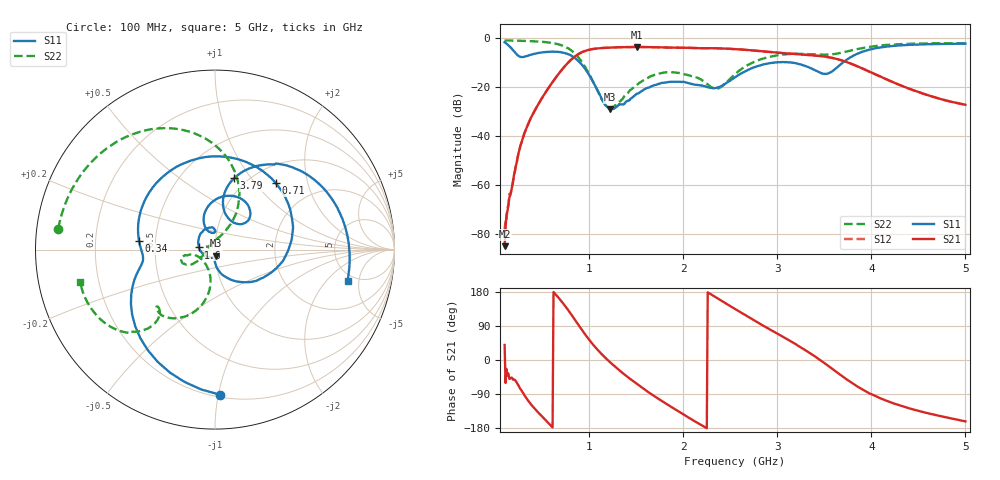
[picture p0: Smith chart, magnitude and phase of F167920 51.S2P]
!  2-Port S-parameters saved by WinCal
! VAR MeasName=S-Parameters (CALIBRATED_DATA) read from VNA (N5242A)
! VAR MeasDate=2016-11-22 9:58:02
! VAR NAME=F167920 51
! VAR FILENAME=F167920 51.S2P
! VAR DATE=2016-11-22 9:58:02
! VAR PHYS_PORTS=1,2
# Hz S DB R 50
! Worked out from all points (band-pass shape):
!   491 points, 100 MHz to 5 GHz, reference 50 ohm
!   highest |S21| = -3.75 dB at 1.51 GHz (marker M1); lowest = -85.1 dB at 100 MHz (marker M2)
!   |S21| within 3 dB of the highest: 881.8 MHz to 3.222 GHz (2.34 GHz wide, 114 % of centre)
!   lowest |S11| = -29.2 dB at 1.22 GHz (marker M3), VSWR 1.07, Z = 50.4 - j3.47 ohm
!   |S11| at or under -10 dB: 897.7 MHz to 3.007 GHz (2.109 GHz wide, 108 % of centre); 3.116 GHz to 3.702 GHz (586 MHz wide, 17.2 % of centre)
!   |S22| runs from -28.7 to -1.1 dB; largest |S21 - S12| = 0.0015
!   S11 on the Smith chart (normalised r, x): 100 MHz: 0.22, -1.01; 340 MHz: 0.40, +0.05; 710 MHz: 1.30, +1.29; 1.6 GHz: 0.83, +0.02; 3.79 GHz: 0.87, +0.83; 5 GHz: 4.33, -3.53
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1e8  -1.84 -88.0  -85.14 39.8  -78.36 -52.7  -1.10 172.4
1.8e8  -4.62 -141.7  -60.63 -47.2  -60.76 -55.6  -1.15 166.3
2.6e8  -7.68 -169.4  -45.45 -73.6  -45.32 -72.4  -1.22 159.9
3.4e8  -7.40 173.5  -36.17 -103.6  -36.14 -103.3  -1.32 153.1
5.5e8  -5.79 104.9  -21.47 -162.2  -21.46 -162.2  -1.84 131.0
7.1e8  -5.99 47.7  -13.00 153.2  -13.00 153.2  -3.13 106.2
8.1e8  -7.32 7.4  -8.85 119.7  -8.86 119.8  -5.21 86.2
9.2e8  -10.83 -37.4  -5.91 80.3  -5.91 80.3  -9.84 65.1
1.07e9  -20.15 -84.8  -4.44 32.1  -4.43 32.1  -20.19 63.7
1.22e9  -29.18 -81.1  -4.02 -5.6  -4.02 -5.6  -28.72 135.7
1.51e9  -22.81 -160.5  -3.75 -63.8  -3.75 -63.8  -19.19 -147.4
1.6e9  -20.79 172.5  -3.78 -79.8  -3.79 -79.8  -16.87 -147.1
1.74e9  -18.81 139.2  -3.91 -103.1  -3.92 -103.2  -14.62 -153.9
2.13e9  -19.18 90.9  -4.22 -162.9  -4.23 -162.9  -16.14 -168.3
2.36e9  -20.38 102.0  -4.31 163.4  -4.31 163.4  -20.83 -134.2
2.55e9  -16.12 112.9  -4.63 134.7  -4.63 134.6  -14.84 -97.9
2.91e9  -10.44 81.0  -5.78 82.2  -5.80 82.2  -7.86 -113.6
3.37e9  -12.68 41.3  -7.13 14.4  -7.14 14.5  -6.76 -135.4
3.54e9  -14.58 64.7  -7.91 -15.1  -7.91 -15.0  -6.89 -133.5
3.79e9  -7.71 75.0  -10.67 -60.0  -10.68 -59.9  -5.13 -129.6
4.19e9  -3.49 37.2  -17.48 -110.4  -17.51 -110.1  -2.86 -142.9
5e9  -2.40 -13.2  -27.38 -162.0  -27.39 -161.6  -2.24 -166.3
